FUNCTION FC 1 : VOID
BEGIN
	L		W#16#1234
	T		MW 0
	CALL		FC 2
END_FUNCTION


FUNCTION FC 2 : VOID
BEGIN
	L		W#16#6789
	T		MW 0
	L		10
	T		LB 0
END_FUNCTION


FUNCTION FC 3 : VOID
BEGIN
	L		1
	T		LB 0
	CALL		FC 2
	__ASSERT==	LB 0,	1
END_FUNCTION


FUNCTION FC 4 : VOID
VAR_INPUT
	INPVAR		: INT
END_VAR
BEGIN
	L		#INPVAR
	__ASSERT==	__ACCU 1,	9976
END_FUNCTION


FUNCTION FC 5 : VOID
VAR_INPUT
	INPVAR2		: INT
END_VAR
BEGIN
	CALL FC 4 (
		INPVAR		:= #INPVAR2,	// This is a parameter
	)
END_FUNCTION


ORGANIZATION_BLOCK OB 1
BEGIN
	CALL		FC 1
	__ASSERT==	MW 0,	W#16#6789
	L		0
	T		MW 0
	__ASSERT==	MW 0,	0
	UC		FC 1
	__ASSERT==	MW 0,	W#16#6789
	L		0
	T		MW 0
	__ASSERT==	MW 0,	0
	SET
	CC		FC 1
	__ASSERT==	MW 0,	W#16#6789
	L		0
	T		MW 0
	__ASSERT==	MW 0,	0
	CLR
	CC		FC 1
	__ASSERT==	MW 0,	0

	// Test localdata stack
	L		255
	T		LB 0
	__ASSERT==	LB 0,	255
	CALL		FC 3
	__ASSERT==	LB 0,	255

	CALL FC 5 (
		INPVAR2		:= 9976,
	)
END_ORGANIZATION_BLOCK
